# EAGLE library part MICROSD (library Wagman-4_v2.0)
Micro-SD / Transflash card holder with SPI pinout For the 3M # 2908-05WB-MG and/or 4UCON #19656 push-push type
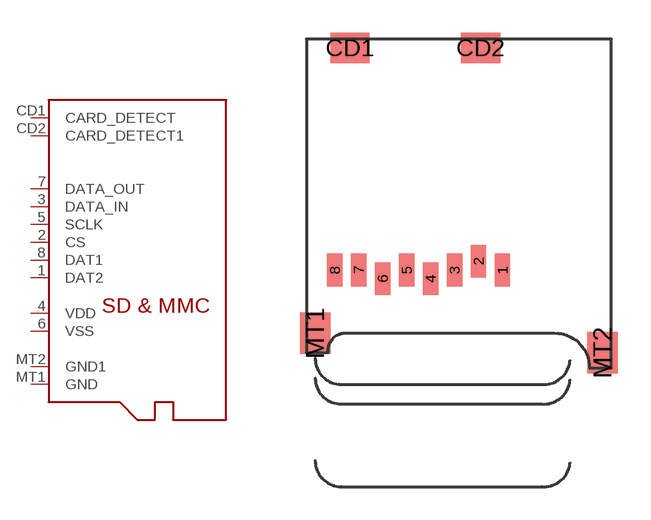
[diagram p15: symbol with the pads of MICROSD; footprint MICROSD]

Designator prefix -

## MICROSD  [MICROSD]
1  DAT2
2  CS  in
3  DATA_IN  in
4  VDD  sup
5  SCLK  in
6  VSS  sup
7  DATA_OUT  out
8  DAT1
CD1  CARD_DETECT  pas
CD2  CARD_DETECT1  pas
MT1  GND  sup
MT2  GND1  sup

## Footprint MICROSD (pad centres in mm)
smd 0.7 x 1.5: 1 9,-10.64; 2 7.9,-10.24; 3 6.8,-10.64; 4 5.7,-11.04; 5 4.6,-10.64; 6 3.5,-11.04; 7 2.4,-10.64; 8 1.3,-10.64
smd 1.8 x 1.4: CD1 2,-0.44; CD2 8,-0.44
smd 1.4 x 1.9: MT1 0.4,-13.54; MT2 13.6,-14.44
